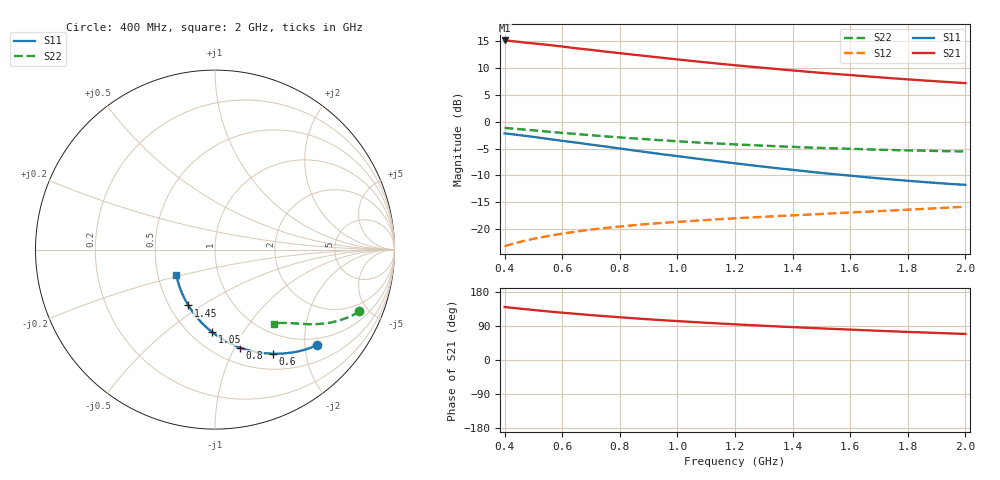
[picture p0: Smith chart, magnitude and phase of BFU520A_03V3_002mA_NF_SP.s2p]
! Filename:  P:\Prog\Test\Noise\ATS_data\Testdata_Net\06 Compressed Noise after Statistics\BFU520A_APG2013_30_A05_03p3V_002mA_NF_CM01_D.sf
! Date/Time: Wed 24/Apr/2013 20:06:16
! BFU520A_APG2013_30_A05_03p3V_1to20mA_NF_CM01_Bias2_R.sf
! Noise Parameter Data File
! BFU520A_APG2013_30_A05_03p3V_1to20mA_NF_CM01
! Date/time: Thu Apr 11 00:04:13 2013
! VAR V_out= 3.301000
! VAR I_out= 2.005000
! VAR V_in= 0.811200
! VAR I_in= 0.021800
! Device data file deembeded for feedlines and parallel
! Original file: \06 Compressed Noise after Statistics\BFU520A_APG2013_30_A05_03p3V_002mA_NF_CM01_R.sf
! Feed-files: PR017V01_150413_Feed1.s2p, PR017V01_150413_Feed2.s2p
! Parallel-file: PR017V01_150413_Par.s2p
# MHz S MA R 50
!  Freq-MHz  S11-mag  S11-arg  S21-mag  S21-arg  S12-mag  S12-arg  S22-mag  S22-arg
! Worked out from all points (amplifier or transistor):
!   37 points, 400 MHz to 2 GHz, reference 50 ohm
!   highest |S21| = 15.1 dB at 400 MHz (marker M1)
!   |S21| within 3 dB of that: start of sweep to 909 MHz
!   unconditionally stable (mu >= 1): nowhere
!   at 500 MHz: K = 0.36, MSG = 18.2 dB, |S12| = -21.8 dB
!   at 1.1 GHz: K = 0.70, MSG = 14.7 dB, |S12| = -18.3 dB
!   at 2 GHz: K = 0.99, MSG = 11.5 dB, |S12| = -15.8 dB
!   lowest NFmin = 0.52 dB at 420 MHz
!   S11 on the Smith chart (normalised r, x): 400 MHz: 0.83, -2.26; 600 MHz: 0.70, -1.46; 800 MHz: 0.66, -1.05; 1.05 GHz: 0.63, -0.74; 1.45 GHz: 0.62, -0.44; 2 GHz: 0.62, -0.19
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400  0.7788 -43.2  5.686 139.9  0.06954 65.7  0.8743 -23.1
420  0.767 -45.2  5.627 138.2  0.07213 64.8  0.8655 -24.0
440  0.7559 -47.0  5.556 136.6  0.07457 63.9  0.8569 -24.8
480  0.7337 -50.6  5.394 133.6  0.07916 62.3  0.8385 -26.4
500  0.7214 -52.5  5.338 132.0  0.08137 61.6  0.8301 -27.1
550  0.6921 -56.8  5.173 128.3  0.0863 59.9  0.807 -28.9
600  0.6631 -61.0  4.992 124.8  0.0909 58.4  0.7863 -30.4
650  0.6385 -64.7  4.802 121.7  0.09522 57.1  0.767 -31.9
700  0.6113 -68.6  4.652 118.5  0.099 56.0  0.7477 -33.2
750  0.5874 -72.1  4.478 115.6  0.1026 55.0  0.7302 -34.4
800  0.563 -75.8  4.333 112.8  0.106 54.1  0.7136 -35.5
850  0.5392 -79.3  4.188 110.0  0.109 53.4  0.698 -36.5
950  0.4963 -85.9  3.917 105.0  0.1145 52.2  0.6694 -38.4
1050  0.4593 -92.1  3.667 100.4  0.1193 51.5  0.6442 -39.9
1100  0.442 -95.2  3.554 98.3  0.1217 51.3  0.6335 -40.6
1200  0.41 -101.1  3.347 94.2  0.1262 51.0  0.6143 -42.1
1300  0.3814 -106.9  3.163 90.3  0.1304 50.8  0.5979 -43.4
1450  0.3447 -115.6  2.916 85.0  0.1365 51.1  0.5757 -45.2
1500  0.3335 -118.3  2.842 83.4  0.1386 51.3  0.5698 -45.8
1650  0.3054 -126.8  2.647 78.6  0.1451 52.0  0.5541 -47.6
1750  0.2894 -132.5  2.527 75.6  0.1495 52.6  0.5445 -48.7
2000  0.2586 -146.7  2.281 68.7  0.1619 54.2  0.5278 -51.7
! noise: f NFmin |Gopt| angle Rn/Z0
400  0.5335  0.5043  16.86  0.2145
460  0.5483  0.4756  21.63  0.2074
600  0.6335  0.4817  27.45  0.2134
800  0.616  0.4504  39.29  0.1764
1000  0.6689  0.4318  49.35  0.1638
1200  0.7191  0.4127  60.52  0.1603
1400  0.754  0.3918  72.21  0.1409
1600  0.7482  0.3692  83.66  0.1228
1800  0.7228  0.3494  103  0.0932
2000  0.7743  0.3322  107.8  0.0964
